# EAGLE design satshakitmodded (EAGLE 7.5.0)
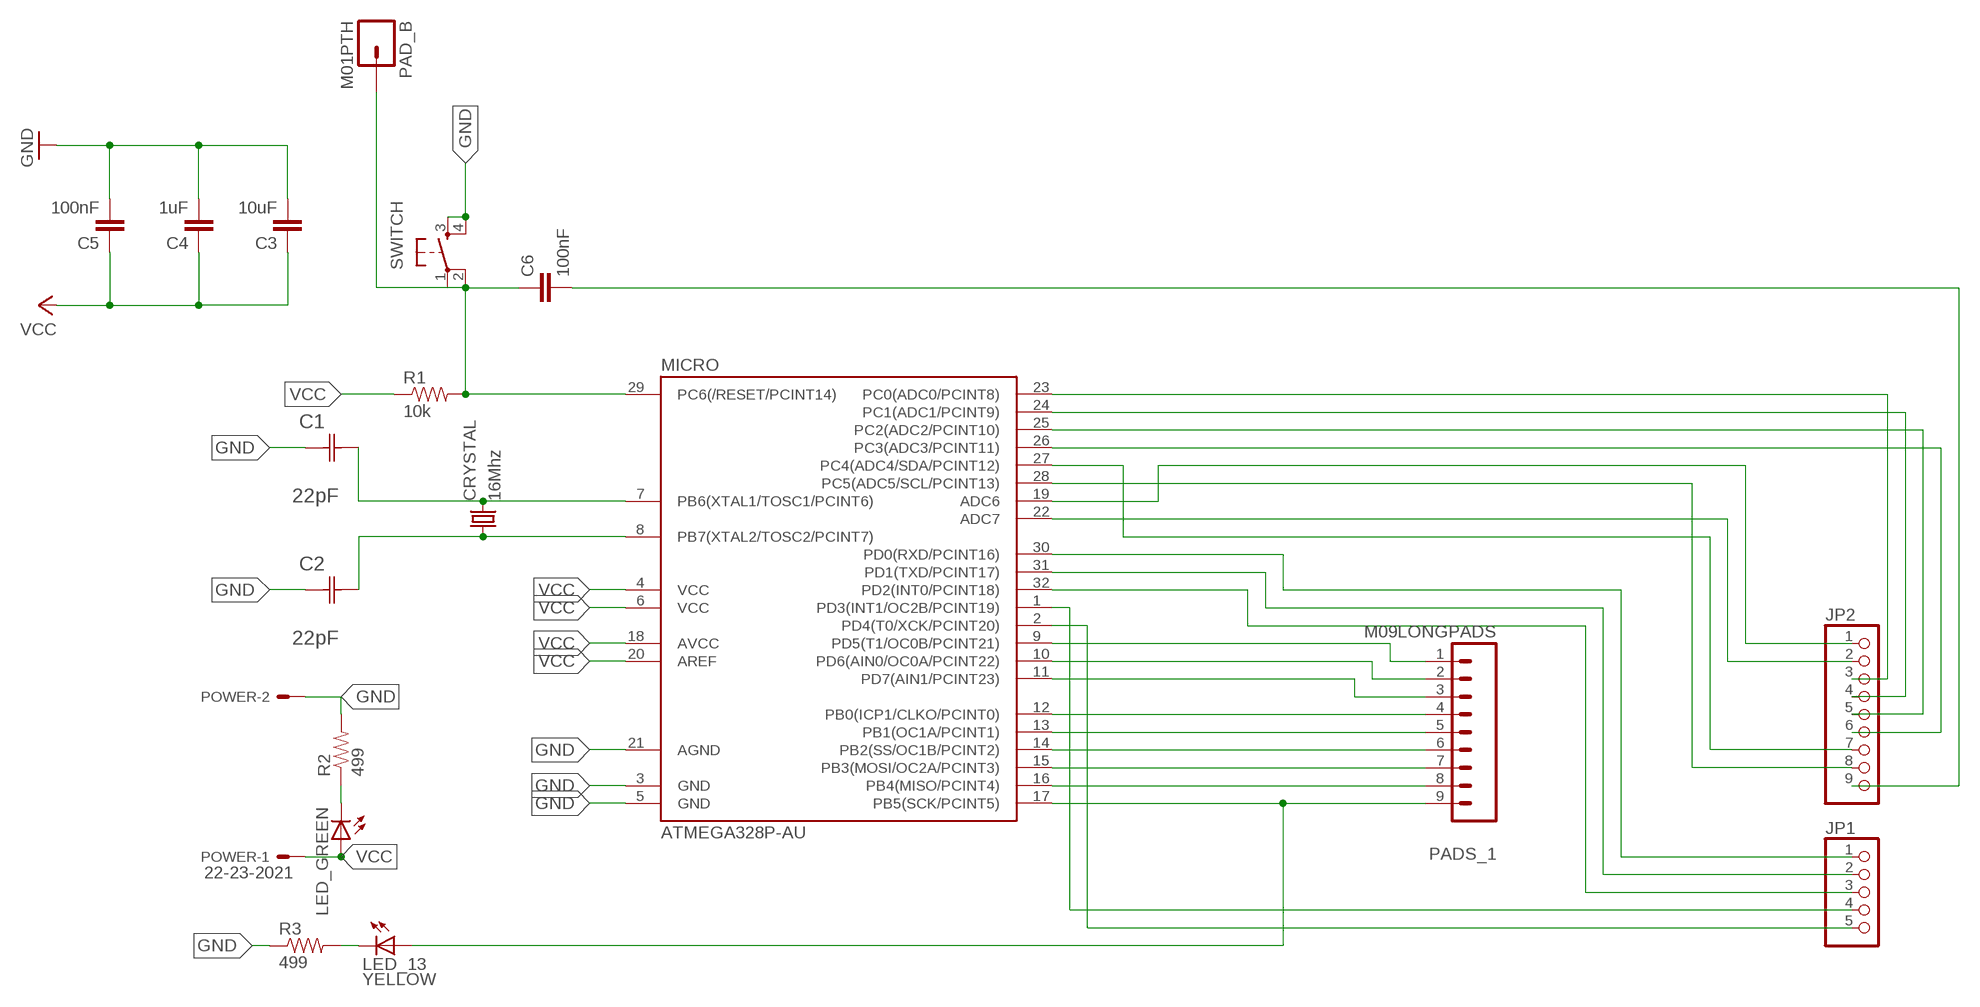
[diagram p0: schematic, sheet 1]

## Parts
C1  22pF  0612ZC225MAT2A  [CAPC3216X178N]
C2  22pF  0612ZC225MAT2A  [CAPC3216X178N]
C3  10uF  CAP1206  [1206]
C4  1uF  CAP1206  [1206]
C5  100nF  CAP1206  [1206]
C6  100nF  CAP1206  [1206]
CRYSTAL  16Mhz  CSM-7X-DU  [CSM-7X-DU]
JP1  PINHD-1X5  [1X05]
JP2  PINHD-1X9  [1X09]
LED_13  YELLOW  LED1206  [1206]
LED_GREEN  LED1206  [1206]
MICRO  ATMEGA328P-AU  ATMEGA48/88/168-AU  [TQFP32-08]
PAD_B  M01PTH  [1X01]
PADS_1  M09LONGPADS  [1X09_LONGPADS]
POWER  22-23-2021  [22-23-2021]
R1  10k  RESISTOR1206  [1206]
R2  499  RESISTOR1206  [1206]
R3  499  RESISTOR1206  [1206]
SWITCH  6MM_SWITCH6MM_SWITCH  [6MM_SWITCH]

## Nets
GND: C1.1(C1) C2.1(C1) C3.2 C4.2 C5.2 MICRO.3(GND) MICRO.5(GND) MICRO.21(AGND) POWER.2 R2.2 R3.1 SWITCH.3(S) SWITCH.4(S1)
N$1: MICRO.9(PD5(T1/OC0B/PCINT21)) PADS_1.1
N$2: C1.2(C2) CRYSTAL.2 MICRO.7(PB6(XTAL1/TOSC1/PCINT6))
N$3: C6.2 JP2.9
N$4: MICRO.10(PD6(AIN0/OC0A/PCINT22)) PADS_1.2
N$5: MICRO.11(PD7(AIN1/PCINT23)) PADS_1.3
N$6: MICRO.12(PB0(ICP1/CLKO/PCINT0)) PADS_1.4
N$7: MICRO.13(PB1(OC1A/PCINT1)) PADS_1.5
N$8: MICRO.14(PB2(SS/OC1B/PCINT2)) PADS_1.6
N$9: C2.2(C2) CRYSTAL.1 MICRO.8(PB7(XTAL2/TOSC2/PCINT7))
N$10: MICRO.15(PB3(MOSI/OC2A/PCINT3)) PADS_1.7
N$11: MICRO.16(PB4(MISO/PCINT4)) PADS_1.8
N$12: LED_13.1(A) MICRO.17(PB5(SCK/PCINT5)) PADS_1.9
N$13: JP2.1 MICRO.19(ADC6)
N$14: JP2.2 MICRO.22(ADC7)
N$15: JP2.3 MICRO.23(PC0(ADC0/PCINT8))
N$16: JP2.4 MICRO.24(PC1(ADC1/PCINT9))
N$17: JP2.5 MICRO.25(PC2(ADC2/PCINT10))
N$18: JP2.6 MICRO.26(PC3(ADC3/PCINT11))
N$19: JP2.7 MICRO.27(PC4(ADC4/SDA/PCINT12))
N$20: JP1.1 MICRO.30(PD0(RXD/PCINT16))
N$21: JP1.2 MICRO.31(PD1(TXD/PCINT17))
N$22: JP1.3 MICRO.32(PD2(INT0/PCINT18))
N$23: JP1.4 MICRO.1(PD3(INT1/OC2B/PCINT19))
N$24: JP1.5 MICRO.2(PD4(T0/XCK/PCINT20))
N$25: JP2.8 MICRO.28(PC5(ADC5/SCL/PCINT13))
N$26: LED_GREEN.2(C) R2.1
N$27: LED_13.2(C) R3.2
N$28: C6.1 MICRO.29(PC6(/RESET/PCINT14)) PAD_B.1 R1.2 SWITCH.1(P) SWITCH.2(P1)
VCC: C3.1 C4.1 C5.1 LED_GREEN.1(A) MICRO.4(VCC) MICRO.6(VCC) MICRO.18(AVCC) MICRO.20(AREF) POWER.1 R1.1

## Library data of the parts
C1 C2 = AVX_By_element14_Batch_1:0612ZC225MAT2A: Capacitor 1206; MPN: 0612ZC225MAT2A; OC_FARNELL: -; OC_NEWARK: 12N3209; SUPPLIER: AVX; TOLERANCE: ±20%; VALUE: 2.2µF; VOLTAGERATING: 10V
C3-C6 = 01_SparkFun:CAP: Capacitor
CRYSTAL = 01_FAB_Hello:CSM-7X-DU: SMD CRYSTAL; OC_FARNELL: unknown; OC_NEWARK: unknown
JP1 = pinhead:PINHD-1X5: PIN HEADER
JP2 = pinhead:PINHD-1X9: PIN HEADER
LED_13 LED_GREEN = 01_FAB_Hello:LED
MICRO = atmega8:ATMEGA48/88/168
PAD_B = 01_SparkFun:M01: Header 1
PADS_1 = 01_SparkFun:M09: Header 9 Standard 9-pin 0.1" header. Use with straight break away headers (SKU : PRT-00116), right angle break away headers (PRT-00553), swiss pins (PRT-00743), machine pins (PRT-00117), and female headers (PRT-00115).
POWER = con-molex:22-23-2021: .100" (2.54mm) Center Header - 2 Pin; MF: MOLEX; MPN: 22-23-2021; OC_FARNELL: 1462926; OC_NEWARK: 25C3832
R1-R3 = 01_SparkFun:RESISTOR: Resistor
SWITCH = 01_FAB_Hello:6MM_SWITCH: OMRON SWITCH

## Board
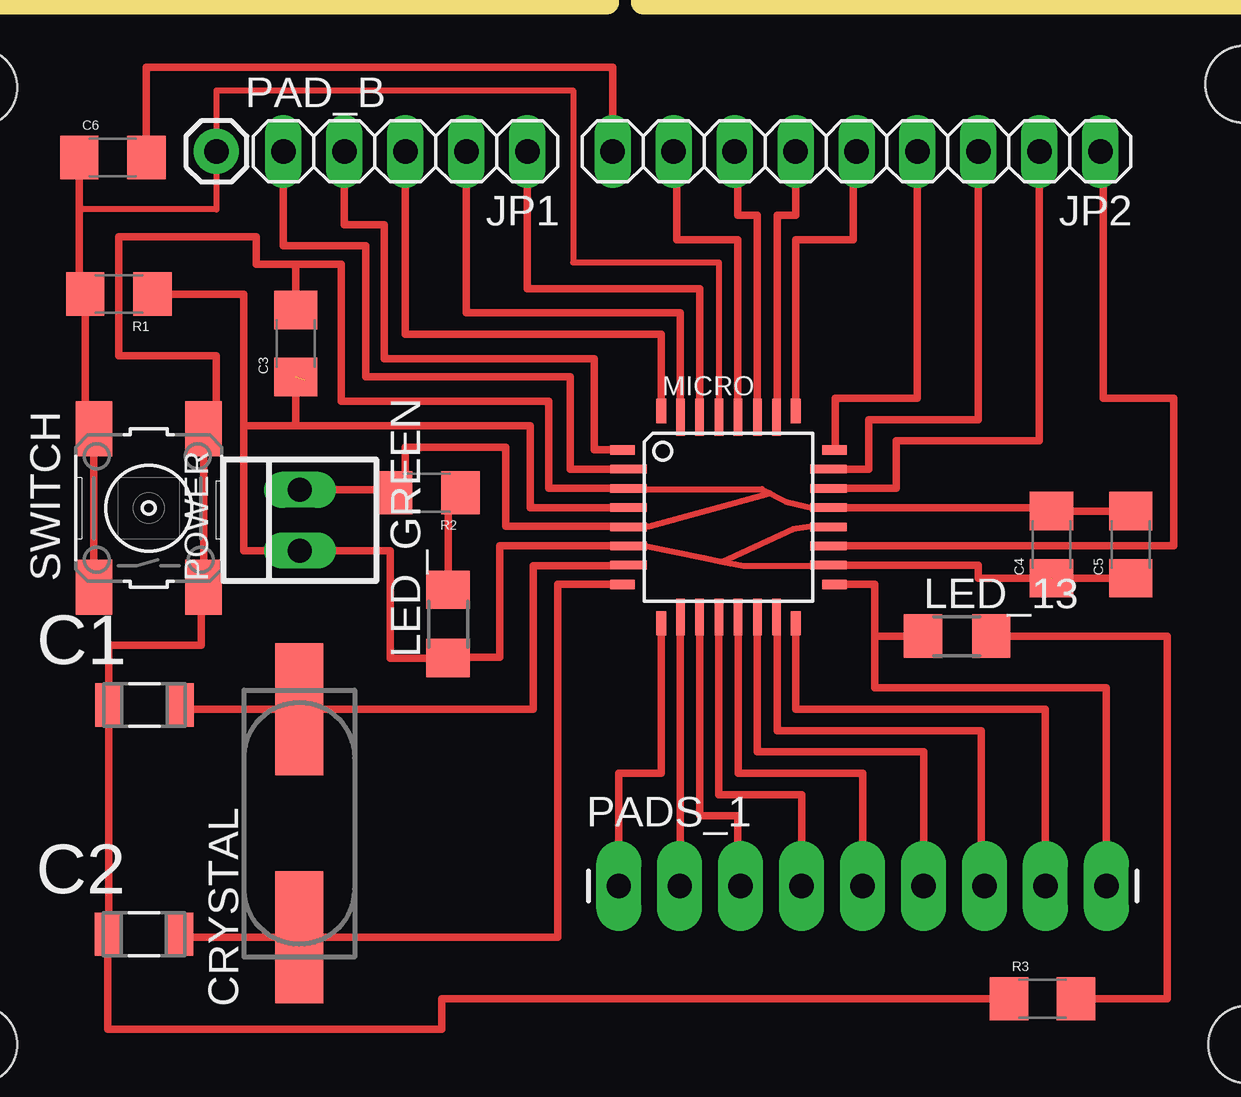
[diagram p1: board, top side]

No outline drawn. Coordinates in mm, seen from the top.
Copper layers (1*16): Top 0.035mm / dielectric 1.5mm / Bottom 0.035mm
Design rules "default": minimum track width 10mil, minimum drill 24mil, track to track 8mil, track to pad 8mil, pad to pad 8mil, via to via 8mil, smd to smd 8mil, copper to edge 40mil, drill to drill 8mil, minimum pad ring 10mil, minimum via ring 8mil, stop-mask expansion 4mil, vias tented up to drill 0mil, thermal gap 10mil
Holes 3.2 mm at 15.75,38.23 68.45,38.35 68.58,-1.65 15.75,-1.65
Milling: 10 lines

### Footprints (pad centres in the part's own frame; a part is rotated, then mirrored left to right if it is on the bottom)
CAPC3216X178N = smd 1.118 x 1.803: 1 -1.499,0; 2 1.499,0
1206 = smd 1.6 x 1.8: 1 -1.4,0; 2 1.4,0
CSM-7X-DU = smd 5.5 x 2: 1 -4.75,0; 2 4.75,0
1X05 = drill 1.016 long: 1 -5.08,0; 2 -2.54,0; 3 0,0; 4 2.54,0; 5 5.08,0
1X09 = drill 1.016 long: 1 -10.16,0; 2 -7.62,0; 3 -5.08,0; 4 -2.54,0; 5 0,0; 6 2.54,0; 7 5.08,0; 8 7.62,0; 9 10.16,0
1206' = smd 1.6 x 1.803: 1 -1.422,0; 2 1.422,0
TQFP32-08 = smd 1.016 x 0.406: 1 -4.42,2.8; 8 -4.42,-2.8; 17 4.42,-2.8; 24 4.42,2.8 | smd 1.524 x 0.356: 2 -4.166,2; 3 -4.166,1.2; 4 -4.166,0.4; 5 -4.166,-0.4; 6 -4.166,-1.2; 7 -4.166,-2; 18 4.166,-2; 19 4.166,-1.2; 20 4.166,-0.4; 21 4.166,0.4; 22 4.166,1.2; 23 4.166,2 | smd 0.406 x 1.016: 9 -2.8,-4.42; 16 2.8,-4.42; 25 2.8,4.42; 32 -2.8,4.42 | smd 0.356 x 1.524: 10 -2,-4.166; 11 -1.2,-4.166; 12 -0.4,-4.166; 13 0.4,-4.166; 14 1.2,-4.166; 15 2,-4.166; 26 2,4.166; 27 1.2,4.166; 28 0.4,4.166; 29 -0.4,4.166; 30 -1.2,4.166; 31 -2,4.166
1X01 = drill 1.016 pad 1.88: 1 0,0
1X09_LONGPADS = drill 1.016 pad 1.88 long: 1 0,0; 2 2.54,0; 3 5.08,0; 4 7.62,0; 5 10.16,0; 6 12.7,0; 7 15.24,0; 8 17.78,0; 9 20.32,0
22-23-2021 = drill 1 long: 1 -1.27,0; 2 1.27,0
6MM_SWITCH = smd 2.286 x 1.524: 1 -3.302,2.286; 2 3.302,2.286; 3 -3.302,-2.286; 4 3.302,-2.286

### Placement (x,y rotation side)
C1  22.66,12.5 0 top
C2  22.63,2.95 0 top
C3  28.96,27.56 90 top
C4  60.45,19.18 90 top
C5  63.75,19.18 90 top
C6  21.34,35.31 0 top
CRYSTAL  29.11,7.57 90 top
JP1  33.53,35.56 180 top
JP2  52.32,35.56 180 top
LED_13  YELLOW  [1206']  56.52,15.37 0 top
LED_GREEN  [1206']  35.31,15.88 90 top
MICRO  46.99,20.32 0 top
PAD_B  25.65,35.56 0 top
PADS_1  42.42,4.95 0 top
POWER  29.13,20.19 90 top
R1  21.59,29.62 180 top
R2  34.42,21.34 180 top
R3  60.07,0.25 0 top
SWITCH  22.83,20.7 90 top

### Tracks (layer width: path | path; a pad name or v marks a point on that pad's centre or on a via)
GND
  Top 0.254: MICRO.3 42.85,21.49 48.38,21.49 | 48.38,21.49 49.4,20.95 50.55,20.7 | 43.43,19.94 43.69,19.94 48.56,21.29 | 48.56,21.29 48.7,21.32 | 48.38,21.49 48.56,21.29
  Top 0.305: MICRO.5 | MICRO.21 | MICRO.5 42.82,19.94 37.72,19.94 37.72,23.24 33.53,23.24 33.53,21.21 33.52,21.21 R2.2 33.52,21.46 POWER.2 | R3.1 35.05,0.25 35.05,-1.02 21.13,-1.02 C2.1 21.16,2.95 C1.1 21.16,14.99 25.02,14.99 25.02,17.4 SWITCH.3 SWITCH.4 25.65,23.88 25.65,27.05 21.59,27.05 21.59,32 27.3,32 27.3,30.86 28.96,30.86 | MICRO.21 60.45,20.72 C4.2 C5.2 | 43.43,19.94 MICRO.5 | MICRO.21 50.55,20.7 | MICRO.3 39.5,21.52 39.5,25.15 30.86,25.15 30.86,30.86 28.96,30.86 | C3.2 28.96,30.86
N$1
  Top 0.305: PADS_1.1 42.42,9.65 44.19,9.65 MICRO.9
N$2
  Top 0.305: MICRO.7 42.82,18.29 38.86,18.29 38.86,12.32 CRYSTAL.2 24.16,12.32 C1.2
N$3
  Top 0.305: C6.2 22.74,39.06 42.16,39.06 JP2.9
N$4
  Top 0.305: PADS_1.2 44.99,4.95 MICRO.10
N$5
  Top 0.305: PADS_1.3 47.37,4.95 47.37,7.87 45.79,7.87 MICRO.11
N$6
  Top 0.305: 46.61,16.15 MICRO.12 46.59,8.76 50.04,8.76 PADS_1.4
N$7
  Top 0.305: PADS_1.5 52.58,9.65 47.39,9.65 MICRO.13
N$8
  Top 0.305: PADS_1.6 55.12,10.54 48.19,10.54 MICRO.14
N$9
  Top 0.305: MICRO.8 39.88,17.53 39.88,2.82 CRYSTAL.1 24.13,2.82 C2.2
N$10
  Top 0.305: PADS_1.7 57.53,4.95 57.53,11.43 49.02,11.43 49.02,15.37 MICRO.15
N$11
  Top 0.305: MICRO.16 49.79,12.32 60.2,12.32 PADS_1.8
N$12
  Top 0.305: PADS_1.9 62.74,13.21 53.09,13.21 53.09,15.37 | LED_13.1 53.09,15.37 | MICRO.17 53.09,17.52 53.09,15.37
N$13
  Top 0.305: MICRO.19 65.53,19.12 65.53,25.27 62.61,25.27 62.61,35.56 JP2.1
N$14
  Top 0.305: MICRO.22 53.98,21.52 53.98,23.5 59.94,23.5 JP2.2
N$15
  Top 0.305: MICRO.23 52.83,22.32 52.83,24.38 57.4,24.38 JP2.3
N$16
  Top 0.305: MICRO.24 51.44,23.12 51.44,25.27 54.86,25.27 JP2.4
N$17
  Top 0.305: MICRO.25 49.78,31.88 52.2,31.88 52.2,35.56 JP2.5
N$18
  Top 0.305: MICRO.26 49.02,24.49 49.02,32.89 49.78,32.89 JP2.6
N$19
  Top 0.305: MICRO.27 48.19,32.89 47.37,32.89 47.37,35.56 JP2.7
N$20
  Top 0.305: MICRO.30 45.79,29.84 38.61,29.84 JP1.1
N$21
  Top 0.305: MICRO.31 44.99,28.83 36.07,28.83 JP1.2
N$22
  Top 0.305: MICRO.32 44.2,27.94 33.53,27.94 JP1.3
N$23
  Top 0.305: MICRO.1 41.4,23.12 41.4,26.92 32.64,26.92 32.64,32.51 30.99,32.51 JP1.4
N$24
  Top 0.305: MICRO.2 40.39,22.32 40.39,26.16 31.88,26.16 31.88,31.62 28.45,31.62 JP1.5
N$25
  Top 0.305: MICRO.28 47.37,24.49 47.37,31.88 44.83,31.88 44.83,35.56 JP2.8
N$26
  Top 0.305: 36.2,21.08 R2.1 35.82,20.95 35.31,20.95 LED_GREEN.2
N$27
  Top 0.305: R3.2 65.28,0.25 65.28,15.37 LED_13.2
N$28
  Top 0.254: MICRO.29 46.59,30.94 40.51,30.94 40.51,38.1 25.65,38.1 PAD_B.1 25.65,33.15 19.94,33.15
  Top 0.305: SWITCH.1 SWITCH.2 | SWITCH.2 20.95,24 | SWITCH.2 20.19,24 R1.2 19.94,29.62 19.94,33.15 C6.1
  Top 0.406: SWITCH.1 20.45,17.4
VCC  (2 unrouted)
  Top 0.254: 43.51,19.13 45.97,18.63 46.72,18.47 | 46.72,18.47 47.62,18.29 51.16,18.29 | MICRO.20 50.55,19.92 50.55,19.94 49.66,19.81 46.72,18.47
  Top 0.305: MICRO.18 | MICRO.20 50.55,19.94 | MICRO.4 38.73,20.72 38.73,24.13 28.96,24.13 | 26.8,24.13 26.8,29.62 R1.1 | 26.8,24.13 26.8,18.92 POWER.1 32.89,18.92 32.89,14.45 LED_GREEN.1 35.31,14.48 37.47,14.48 37.47,19.12 MICRO.6 43.51,19.13 | 51.16,18.29 MICRO.18 | MICRO.18 57.4,18.32 57.4,17.78 C4.1 | 29.34,26.03 29.34,25.91 | 26.8,24.13 28.96,24.13 | 28.96,24.13 C3.1 | C4.1 C5.1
